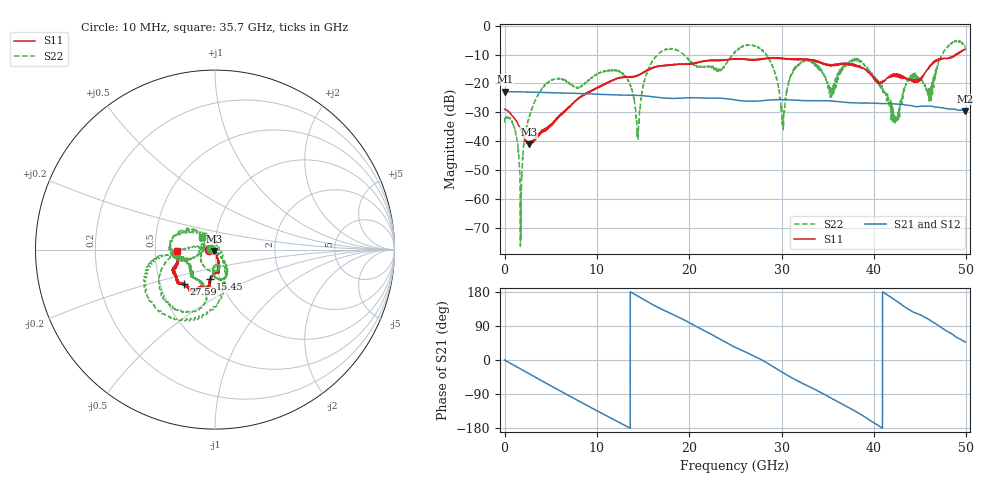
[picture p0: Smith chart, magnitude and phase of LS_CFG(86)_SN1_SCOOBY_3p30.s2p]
!Keysight Technologies,N5245B,MY58422026,A.13.80.08
!Date: Thursday, March 19, 2020 23:54:02
!Correction: S11(Full 2 Port(1,2))
!S21(Full 2 Port(1,2))
!S12(Full 2 Port(1,2))
!S22(Full 2 Port(1,2))
!S2P File: Measurements: S11, S21, S12, S22:
# Hz S DB R 50.0
!freq dBS11 angS11 dBS21 angS21 dBS12 angS12 dBS22 angS22
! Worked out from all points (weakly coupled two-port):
!   4991 points, 10 MHz to 49.91 GHz, reference 50 ohm
!   highest |S21| = -22.80 dB at 20 MHz (marker M1); lowest = -29.5 dB at 49.91 GHz (marker M2)
!   lowest |S11| = -41.1 dB at 2.63 GHz (marker M3), VSWR 1.02, Z = 49.5 - j0.727 ohm
!   |S11| at or under -10 dB: start of sweep to 48.8 GHz; 48.80034 GHz to 48.88179 GHz (81.45 MHz wide, 0.167 % of centre); 48.9521 GHz to 48.9802 GHz (28.11 MHz wide, 0.0574 % of centre)
!   |S22| runs from -76.4 to -5.1 dB; largest |S21 - S12| = 0.0007
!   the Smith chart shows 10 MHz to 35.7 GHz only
!   S11 on the Smith chart (normalised r, x): 10 MHz: 0.93, -0.01; 15.45 GHz: 0.90, -0.30; 27.59 GHz: 0.66, -0.27; 35.7 GHz: 0.65, -0.01
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1e7  -28.97 -175.6  -22.80 -0.3  -22.78 -0.3  -33.56 177.7
2e7  -28.89 -178.8  -22.80 -0.4  -22.80 -0.4  -32.44 -179.3
1.07e9  -32.10 -178.5  -22.88 -14.8  -22.86 -14.7  -35.32 -129.1
1.77e9  -35.98 -166.7  -22.91 -24.3  -22.91 -24.3  -64.00 16.3
2.63e9  -41.08 -123.8  -22.99 -36.0  -22.98 -36.0  -32.08 129.6
4.87e9  -34.63 -68.6  -23.20 -66.2  -23.19 -66.2  -19.32 -129.2
8.33e9  -24.65 -74.1  -23.51 -112.2  -23.50 -112.1  -20.94 -89.9
1.261e10  -17.87 -80.3  -24.02 -166.9  -24.02 -166.8  -16.14 -65.0
1.444e10  -17.21 -92.0  -24.15 168.6  -24.14 168.7  -38.75 -112.8
1.545e10  -15.55 -99.8  -24.41 154.4  -24.40 154.5  -15.81 177.0
1.665e10  -14.10 -99.1  -24.84 138.5  -24.84 138.6  -9.80 -157.7
2.496e10  -11.55 -122.2  -25.68 33.6  -25.67 33.8  -9.23 -168.6
2.759e10  -11.82 -132.5  -26.06 3.6  -26.06 3.8  -7.77 -109.6
3.014e10  -11.40 -142.4  -25.68 -33.1  -25.69 -32.8  -32.19 28.8
3.125e10  -11.50 -147.6  -25.75 -48.7  -25.76 -48.4  -15.44 137.0
3.328e10  -11.87 -156.3  -25.98 -74.0  -25.98 -73.5  -12.32 -173.6
3.57e10  -13.41 -177.1  -26.20 -104.9  -26.14 -104.4  -20.01 142.1
3.817e10  -14.22 172.1  -26.76 -137.8  -26.72 -137.9  -11.43 -172.8
4.16e10  -17.65 106.7  -27.01 169.5  -27.03 169.5  -25.56 73.7
4.245e10  -16.85 104.2  -27.14 155.6  -27.16 155.5  -33.00 -174.3
4.39e10  -18.69 77.5  -27.64 131.7  -27.66 131.9  -17.74 -32.6
4.991e10  -8.18 -13.4  -29.53 47.7  -29.55 47.7  -7.31 -14.6
